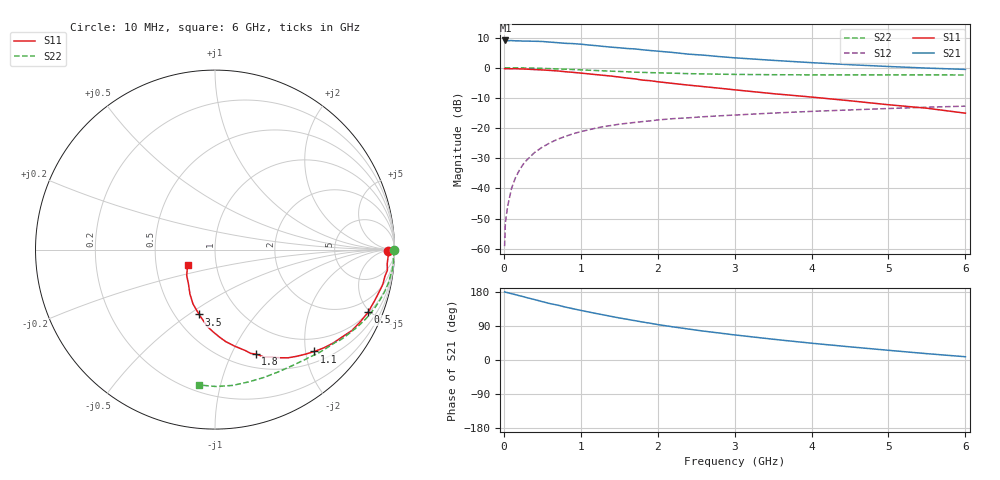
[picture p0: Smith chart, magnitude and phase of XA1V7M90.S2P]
! SIEMENS Discrete & RF Semiconductors
! BFY180
! Si NPN RF Bipolar Junction Transistor in MICRO-X
! VCE = 1.75 V  IC = 0.9 mA
! Common Emitter S-Parameters:  May  1997
# GHz  S  MA  R  50
!  f  S11  S21  S12  S22
! GHz  MAG  ANG  MAG  ANG  MAG  ANG  MAG  ANG
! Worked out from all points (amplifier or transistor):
!   36 points, 10 MHz to 6 GHz, reference 50 ohm
!   highest |S21| = 9.1 dB at 20 MHz (marker M1)
!   |S21| within 3 dB of that: start of sweep to 1.769 GHz
!   unconditionally stable (mu >= 1): 3.759 GHz to end of sweep
!   at 250 MHz: K = 0.07, MSG = 20.4 dB, |S12| = -32.0 dB
!   at 1.4 GHz: K = 0.51, MSG = 13.0 dB, |S12| = -19.1 dB
!   at 6 GHz: K = 1.07, MAG = 4.4 dB, |S12| = -12.7 dB
!   S11 on the Smith chart (normalised r, x): 10 MHz: 53, -13; 500 MHz: 1.05, -4.85; 1.1 GHz: 0.71, -2.18; 1.8 GHz: 0.65, -1.24; 3.5 GHz: 0.65, -0.55; 6 GHz: 0.72, -0.13
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0.01  0.9648 -0.5  2.805 179.7  0.0011 75.5  0.9973 -0.2
0.02  0.9643 -1.0  2.839 178.9  0.0027 97.6  0.9999 -0.6
0.05  0.9657 -2.0  2.808 177.7  0.0051 88.9  0.9971 -1.4
0.1  0.9628 -4.6  2.828 175.0  0.01 88.5  0.9942 -2.7
0.15  0.9673 -6.9  2.797 172.5  0.0149 85.9  0.9969 -4.1
0.25  0.9552 -11.5  2.768 167.4  0.025 82.7  0.9943 -6.8
0.3  0.9497 -13.1  2.769 164.4  0.0296 80.7  0.9891 -8.1
0.5  0.9212 -22.3  2.731 154.0  0.0483 74.3  0.977 -13.1
0.6  0.9042 -26.4  2.666 148.8  0.0569 71.3  0.9672 -15.5
0.9  0.8396 -38.3  2.517 135.3  0.0805 63.0  0.9352 -22.5
1.1  0.7931 -45.7  2.389 126.8  0.0934 57.9  0.9118 -26.8
1.2  0.7699 -49.2  2.327 122.7  0.1001 55.5  0.9008 -28.8
1.5  0.7022 -59.1  2.148 111.0  0.116 49.5  0.8686 -34.4
1.8  0.6247 -68.7  1.99 100.3  0.128 45.0  0.8388 -39.3
2.2  0.5497 -78.4  1.793 87.4  0.1433 38.8  0.8131 -45.5
2.6  0.4864 -87.3  1.618 76.1  0.1543 34.7  0.7908 -51.0
3  0.4313 -95.6  1.463 66.2  0.1645 30.6  0.7769 -56.3
3.5  0.3721 -103.8  1.328 54.8  0.1774 26.5  0.7671 -62.7
4  0.3269 -112.0  1.216 44.3  0.1892 22.4  0.7626 -69.1
4.5  0.2837 -119.5  1.125 34.7  0.2 18.6  0.7606 -75.7
5.5  0.2134 -137.6  0.988 16.7  0.222 10.5  0.7628 -89.6
6  0.1766 -150.0  0.94 8.6  0.2309 6.3  0.7594 -96.7
